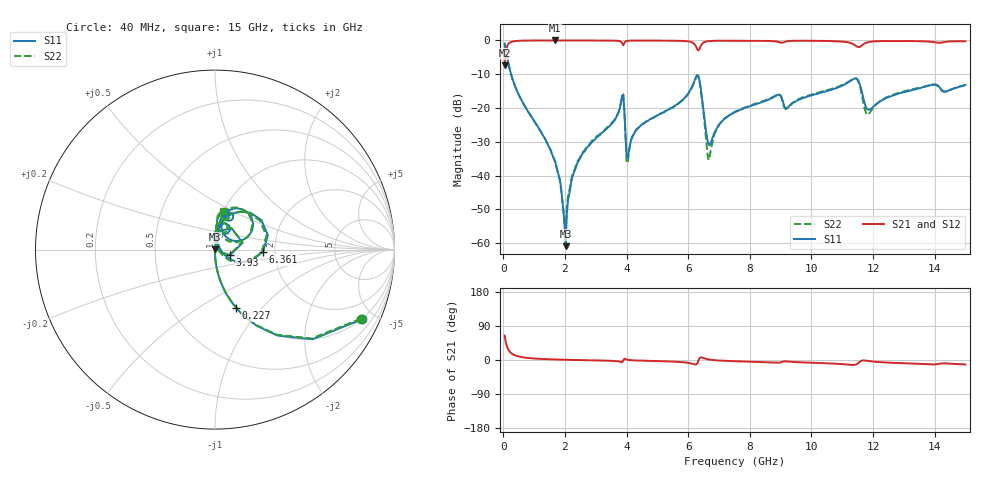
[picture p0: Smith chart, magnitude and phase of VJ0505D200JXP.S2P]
! VJ0505D200JXP
! MLCC placed on 25 mil thick microstrip substrate in series configuraton.
! DATE 06/29/2018  09:06
! CORRECTED  DATA
# GHz  S  MA  R  50.00
!  FREQ  S11M  S11A  S21M  S21A  S12M  S12A  S22M  S22A
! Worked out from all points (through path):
!   401 points, 40 MHz to 15 GHz, reference 50 ohm
!   highest |S21| = -0.01 dB at 1.686 GHz (marker M1); lowest = -7.3 dB at 40 MHz (marker M2)
!   group delay of S21, straight-line fit = 3.29 ps
!   lowest |S11| = -60.9 dB at 2.022 GHz (marker M3), VSWR 1.00, Z = 50 + j0.0816 ohm
!   |S11| at or under -10 dB: 250.2 MHz to end of sweep
!   |S22| runs from -56.0 to -0.9 dB; largest |S21 - S12| = 0.0024
!   S11 on the Smith chart (normalised r, x): 40 MHz: 0.98, -4.21; 227 MHz: 1.00, -0.73; 3.93 GHz: 1.18, -0.07; 6.361 GHz: 1.73, -0.05; 15 GHz: 1.01, +0.45
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0.04  0.9052 -25.4  0.4296 64.5  0.4299 64.5  0.8986 -25.4
0.227  0.3454 -70.1  0.9387 20.2  0.939 20.3  0.3422 -69.9
1.6856  0.01575 -89.1  0.999 1.4  0.9989 1.5  0.01571 -93.8
2.0222  0.0009017 64.8  0.9988 0.6  0.9984 0.7  0.001579 120.7
2.2466  0.009771 86.1  0.9973 0.2  0.998 0.3  0.0105 95.4
2.5458  0.02029 86.2  0.9969 -0.3  0.9974 -0.3  0.02118 90.7
3.8174  0.1192 66.9  0.9579 -5.3  0.9584 -5.3  0.1206 69.6
3.9296  0.08851 -20.7  0.918 3.3  0.9185 3.3  0.08645 -20.0
4.0044  0.01846 6.8  0.9813 1.2  0.9815 1.3  0.01532 12.0
4.0792  0.02375 67.3  0.991 0.0  0.9915 0.1  0.02286 78.8
4.341  0.04871 83.6  0.9954 -1.4  0.9956 -1.4  0.04927 89.8
5.0516  0.07984 83.6  0.9939 -3.0  0.994 -3.0  0.07913 88.7
6.1736  0.2317 61.7  0.9092 -10.9  0.9098 -10.9  0.2281 63.3
6.3606  0.2681 -2.6  0.7377 3.7  0.7385 3.7  0.2588 -3.8
6.6598  0.02892 12.4  0.9767 1.5  0.9768 1.5  0.017 18.7
7.0338  0.05927 77.0  0.9908 -1.5  0.991 -1.5  0.05906 88.9
7.52  0.0872 80.7  0.9915 -3.2  0.9923 -3.2  0.08806 89.7
10.0258  0.1549 80.7  0.9871 -7.2  0.9882 -7.2  0.1593 86.3
11.4096  0.2742 51.9  0.8526 -12.7  0.8527 -12.8  0.2727 52.3
11.8584  0.09425 47.9  0.947 -2.6  0.9472 -2.6  0.08043 59.0
12.5316  0.1466 75.2  0.9808 -7.0  0.9812 -7.0  0.1498 85.6
15  0.2186 76.0  0.9709 -11.8  0.9717 -11.8  0.2197 79.0
